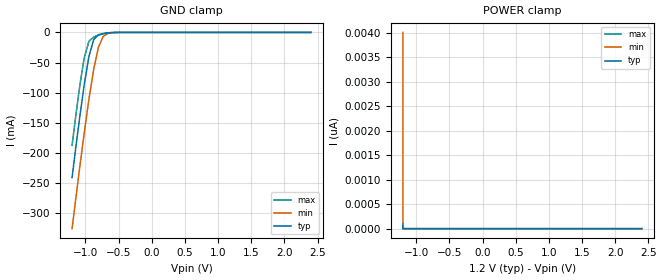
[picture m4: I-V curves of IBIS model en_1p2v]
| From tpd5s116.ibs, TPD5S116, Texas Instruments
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[Model]   en_1p2v
Model_type   Input
Vinl = 0.4
Vinh = 1
|   typ   min   max
|   (nom PVT)   (slow PVT)   (fast PVT)
C_comp   0.787p   0.739p   0.858p
| Where nom  PVT is Nominal Process, 1.2V, 27C
|   Fast PVT is Strong Process,  1.3V, -40C
|   Slow PVT is Weak Process,   1.1V, 125C
[Voltage Range]   1.2   1.1   1.3
[Temperature Range]   27   125   -40
[Power Clamp Reference]   1.2   1.1   1.3
[GND Clamp Reference]   -0   -0   -0
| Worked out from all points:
|   GND clamp passes 1 mA (typ) near -0.67 V on its own axis
[GND Clamp]
|   Voltage   I(typ)   I(min)   I(max)
-1.2V     -240.4mA   -325.2mA   -186.9mA
-1.124V   -173.7mA   -257.7mA   -121.1mA
-1.08V    -136.2mA   -219.2mA   -85.22mA
-1.018V   -87.42mA   -167.4mA   -42.46mA
-946.2mV  -39.58mA   -110.6mA   -14.64mA
-874.4mV  -11.84mA   -60.99mA   -7.757mA
-802.5mV  -4.081mA   -24.24mA   -4.462mA
-730.5mV  -1.866mA   -6.509mA   -2.129mA
-658.5mV  -756.3uA   -1.658mA   -745.3uA
-514.5mV  -59.1uA    -147.6uA   -35.49uA
2.4V      0A         0A         0A
[POWER Clamp]
|   Voltage   I(typ)   I(min)   I(max)
-1.2V     105.9pA    4.006nA    45.24pA
-1.2V     0A         0A         0A
-1.2V     0A         0A         0A
2.4V      0A         0A         0A
